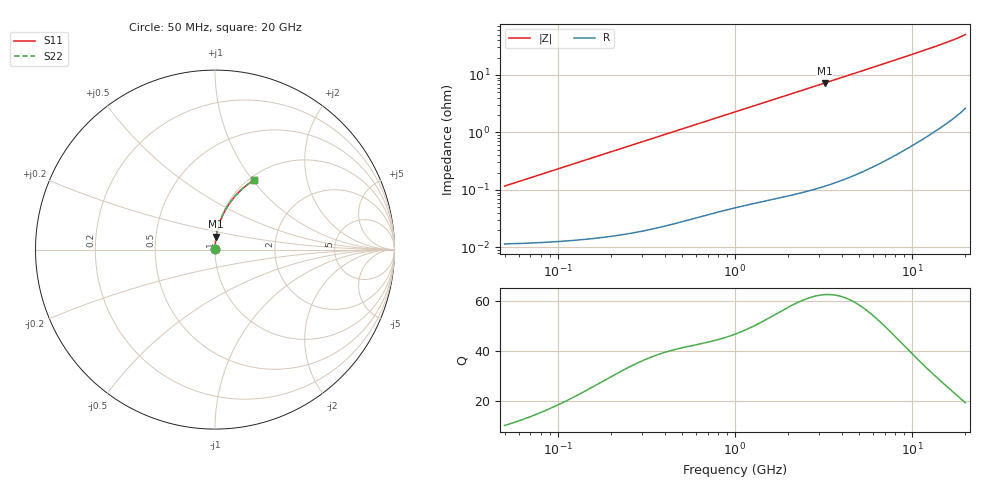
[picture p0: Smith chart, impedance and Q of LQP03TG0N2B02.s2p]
!Murata Part Number: LQP03TG0N2B02
!These Parameters are Measured in Series Mode Connection
!  o--[Z]--o
!Port1  Port2
!  o-------o
!Freq. Start=50[MHz] Stop=20[GHz], 401[Steps]
# Hz S RI R 50
!Freq.(Hz) S11(Real) S11(Imag) S21(Real) S21(Imag) S12(Real) S12(Imag) S22(Real) S22(Imag)
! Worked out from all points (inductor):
!   401 points, 50 MHz to 20 GHz, reference 50 ohm
!   read as one part in series: L = 369 pH near 51.52 MHz
!   highest Q = 62.4 at 3.217 GHz (marker M1), where L = 358 pH
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5e7  0.000116 0.00116  0.9999 -0.00116  0.9999 -0.00116  0.000116 0.00116
5.152053e7  0.000117 0.00119  0.9999 -0.00119  0.9999 -0.00119  0.000117 0.00119
1.364002e8  0.000146 0.00315  0.9999 -0.00315  0.9999 -0.00315  0.000146 0.00315
3.721004e8  0.000295 0.00854  0.9997 -0.00854  0.9997 -0.00854  0.000295 0.00854
6.380365e8  0.000553 0.0146  0.9994 -0.0146  0.9994 -0.0146  0.000553 0.0146
1e9  0.001 0.0227  0.999 -0.0227  0.999 -0.0227  0.001 0.0227
1.714689e9  0.0022 0.0386  0.9978 -0.0386  0.9978 -0.0386  0.0022 0.0386
2.728004e9  0.00474 0.061  0.9953 -0.061  0.9953 -0.061  0.00474 0.061
3.216634e9  0.00635 0.0718  0.9937 -0.0718  0.9937 -0.0718  0.00635 0.0718
4.026975e9  0.00957 0.0896  0.9904 -0.0896  0.9904 -0.0896  0.00957 0.0896
5.041459e9  0.0146 0.1116  0.9854 -0.1116  0.9854 -0.1116  0.0146 0.1116
6.125241e9  0.0211 0.1348  0.9789 -0.1348  0.9789 -0.1348  0.0211 0.1348
7.442007e9  0.0307 0.1624  0.9693 -0.1624  0.9693 -0.1624  0.0307 0.1624
8.774992e9  0.0421 0.1895  0.9579 -0.1895  0.9579 -0.1895  0.0421 0.1895
1.019291e10  0.0562 0.2175  0.9438 -0.2175  0.9438 -0.2175  0.0562 0.2175
1.166392e10  0.0727 0.2455  0.9273 -0.2455  0.9273 -0.2455  0.0727 0.2455
1.334722e10  0.0942 0.276  0.9058 -0.276  0.9058 -0.276  0.0942 0.276
1.504638e10  0.1187 0.3053  0.8813 -0.3053  0.8813 -0.3053  0.1187 0.3053
1.670968e10  0.1459 0.3328  0.8541 -0.3328  0.8541 -0.3328  0.1459 0.3328
1.800918e10  0.17 0.3536  0.83 -0.3536  0.83 -0.3536  0.17 0.3536
1.940974e10  0.2003 0.376  0.7997 -0.376  0.7997 -0.376  0.2003 0.376
2e10  0.2151 0.3856  0.7849 -0.3856  0.7849 -0.3856  0.2151 0.3856
